(* Logix 5000 AddOnInstructionDefinition export EipIoDataMapping_GS30A_CM_EIP1; software revision 37.00 *)

ADD_ON_INSTRUCTION EipIoDataMapping_GS30A_CM_EIP1   (* revision 1.0, vendor Automationdirect.com *)
// This Add-On Instruction unpacks raw Input Data (T->O) from an array and maps this data into meaningful drive related status tags for the user. Likewise, the AOI also maps meaningful drive related command tags and packs the data into the raw Output Data (O->T) array.
// The purpose of the Add-On Instruction is to simplify the mapping (packing/unpacking) of the raw Input/Output Data. For operation of the drive, the user must provide their own logic.
// Revision note:
// Created in v37.00.00
// Version: 1.0
// - Initial version of the new Add-On Instruction format.
// 2025/06/27
VAR_IN_OUT
   mod_EipInputData : _0294:GS30A_CM_EIP1_E8411017:I:0; {required}   // Module defined using SINT data type
   mod_EipOutputData : _0294:GS30A_CM_EIP1_E771E08B:O:0; {required}   // Module defined using SINT data type
END_VAR
VAR_INPUT
   cmd_Run : BOOL; {visible}
   cmd_Stop : BOOL; {visible}
   cmd_Jog : BOOL; {visible}
   cmd_DirectionCommand : BOOL; {visible}   // False = Fwd; True = Rev
   cmd_NthAccelDecel : SINT; {visible}
   cmd_NthStepSpeedFrequency : SINT; {visible}
   cmd_EnableBitFunction_6_11 : BOOL; {visible}   // Enables the Nth Accel/Decel and Nth Step Speed Freq functionality
   cmd_FrequencyCommand : REAL; {visible}   // xx.xx Hz
   cmd_ExternalFaultTrigger : BOOL; {visible}
   cmd_ResetCommand : BOOL; {visible}
   cmd_ExternalInterruption : BOOL; {visible}
END_VAR
VAR_OUTPUT
   sts_WarningCode : SINT; {access Read Only, visible}
   sts_FaultCode : SINT; {access Read Only, visible}
   sts_Stop : BOOL; {access Read Only, visible}
   sts_DecelDuringStop : BOOL; {access Read Only, visible}
   sts_Standby : BOOL; {access Read Only, visible}
   sts_Run : BOOL; {access Read Only, visible}
   sts_Fwd : BOOL; {access Read Only, visible}
   sts_TransitioningRevToFwd : BOOL; {access Read Only, visible}
   sts_TransitioningFwdToRev : BOOL; {access Read Only, visible}
   sts_Rev : BOOL; {access Read Only, visible}
   sts_JogActive : BOOL; {access Read Only, visible}
   sts_FreqFromComm : BOOL; {access Read Only, visible}
   sts_FreqFromAnalogOrDiscrete : BOOL; {access Read Only, visible}
   sts_CommandFromCommKeypad : BOOL; {access Read Only, visible}
   sts_ParametersLocked : BOOL; {access Read Only, visible}
   sts_DriveStopped : BOOL; {access Read Only, visible}
   sts_DriveRunning : BOOL; {access Read Only, visible}
   sts_FreqCommand_PIDSetpoint : REAL; {access Read Only, visible}
   sts_OutputFrequency : REAL; {access Read Only, visible}   // xx.xx Hz
   sts_OutputCurrent : REAL; {access Read Only, visible}
   sts_DcBusVoltage : REAL; {access Read Only, visible}
   sts_OutputVoltage : REAL; {access Read Only, visible}   // xxx.x
   sts_MultiSpeed_PIDStepNumber : INT; {access Read Only, visible}
   sts_MaxOutputTorque : INT; {access Read Only, visible}
   sts_DigitalInputCounterValue : INT; {access Read Only, visible}
   sts_PowerFactorAngle : REAL; {access Read Only, visible}   // xxx.x degrees
   sts_OutputTorque : REAL; {access Read Only, visible}
   sts_ActualMotorSpeed : INT; {access Read Only, visible}   // xxxx RPM
   sts_EncoderFeedbackCounts : INT; {access None, visible}   // 0 to 65535
   sts_PulseCommandPositionCounts : INT; {access None, visible}   // 0 to 65535
   sts_PowerOutput : INT; {access Read Only, visible}   // xxxx kW (implied decimal)
END_VAR
VAR
   loc_iTemp : INT; {access None}   // Local INT for temporary data manipulation
END_VAR

ROUTINE Logic   (* ladder *)
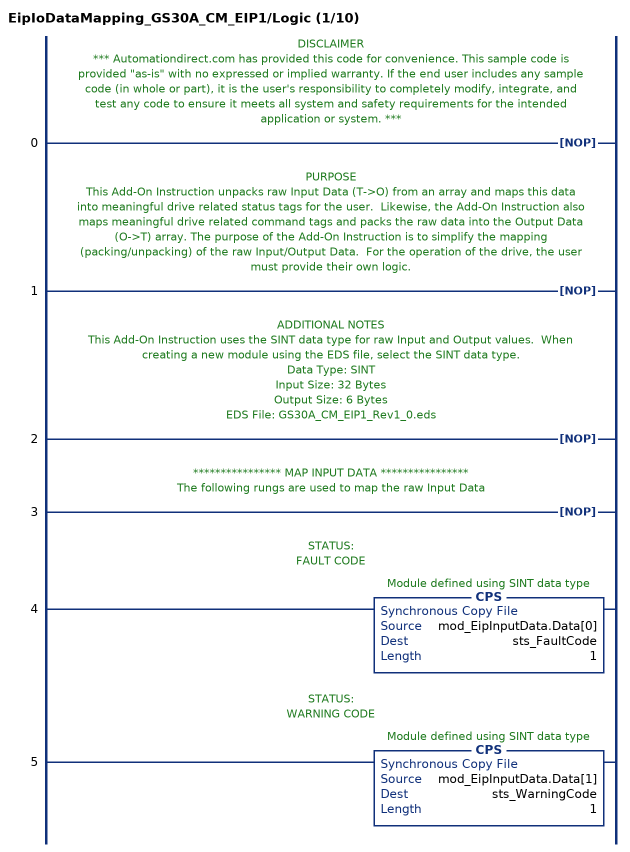
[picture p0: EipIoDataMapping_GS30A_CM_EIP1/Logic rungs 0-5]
   // DISCLAIMER
   // *** Automationdirect.com has provided this code for convenience. This sample code is provided "as-is" with no expressed or implied warranty. If the end user includes any sample code (in whole or part), it is the user's responsibility to completely modify, integrate, and test any code to ensure it meets all system and safety requirements for the intended application or system. ***
   0: NOP();
   // PURPOSE
   // This Add-On Instruction unpacks raw Input Data (T->O) from an array and maps this data into meaningful drive related status tags for the user.  Likewise, the Add-On Instruction also maps meaningful drive related command tags and packs the raw data into the Output Data (O->T) array. The purpose of the Add-On Instruction is to simplify the mapping (packing/unpacking) of the raw Input/Output Data.  For the operation of the drive, the user must provide their own logic.
   1: NOP();
   // ADDITIONAL NOTES
   // This Add-On Instruction uses the SINT data type for raw Input and Output values.  When creating a new module using the EDS file, select the SINT data type.
   // Data Type: SINT
   // Input Size: 32 Bytes
   // Output Size: 6 Bytes
   // EDS File: GS30A_CM_EIP1_Rev1_0.eds
   2: NOP();
   // **************** MAP INPUT DATA ****************
   // The following rungs are used to map the raw Input Data
   3: NOP();
   // STATUS:
   // FAULT CODE
   4: CPS(mod_EipInputData.Data[0],sts_FaultCode,1);
   // STATUS:
   // WARNING CODE
   5: CPS(mod_EipInputData.Data[1],sts_WarningCode,1);
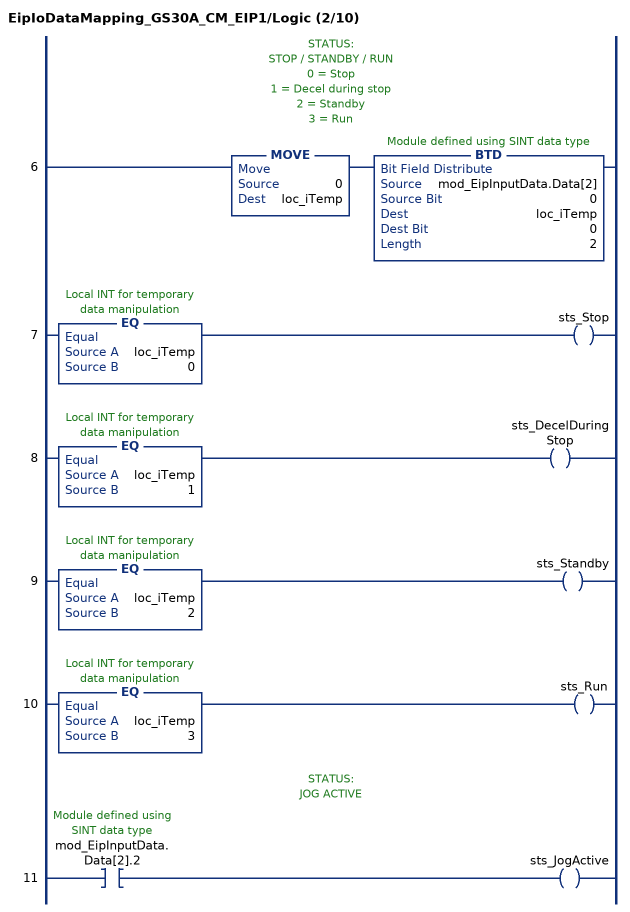
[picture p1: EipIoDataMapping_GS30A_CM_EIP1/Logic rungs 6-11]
   // STATUS:
   // STOP / STANDBY / RUN
   // 0 = Stop
   // 1 = Decel during stop
   // 2 = Standby
   // 3 = Run
   6: MOVE(0,loc_iTemp)BTD(mod_EipInputData.Data[2],0,loc_iTemp,0,2);
   7: EQ(loc_iTemp,0)OTE(sts_Stop);
   8: EQ(loc_iTemp,1)OTE(sts_DecelDuringStop);
   9: EQ(loc_iTemp,2)OTE(sts_Standby);
   10: EQ(loc_iTemp,3)OTE(sts_Run);
   // STATUS:
   // JOG ACTIVE
   11: XIC(mod_EipInputData.Data[2].2)OTE(sts_JogActive);
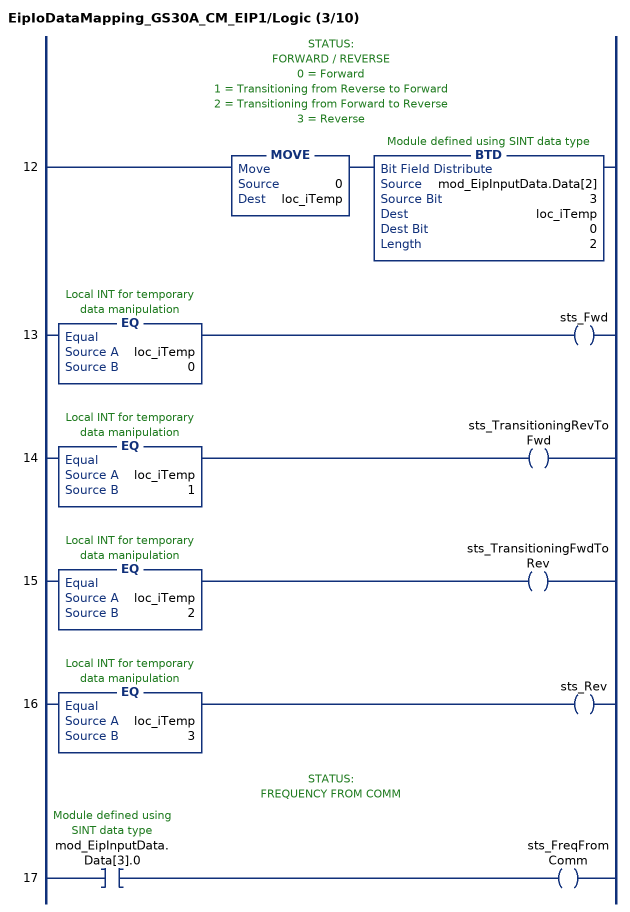
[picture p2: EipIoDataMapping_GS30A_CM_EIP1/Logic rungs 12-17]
   // STATUS:
   // FORWARD / REVERSE
   // 0 = Forward
   // 1 = Transitioning from Reverse to Forward
   // 2 = Transitioning from Forward to Reverse
   // 3 = Reverse
   12: MOVE(0,loc_iTemp)BTD(mod_EipInputData.Data[2],3,loc_iTemp,0,2);
   13: EQ(loc_iTemp,0)OTE(sts_Fwd);
   14: EQ(loc_iTemp,1)OTE(sts_TransitioningRevToFwd);
   15: EQ(loc_iTemp,2)OTE(sts_TransitioningFwdToRev);
   16: EQ(loc_iTemp,3)OTE(sts_Rev);
   // STATUS:
   // FREQUENCY FROM COMM
   17: XIC(mod_EipInputData.Data[3].0)OTE(sts_FreqFromComm);
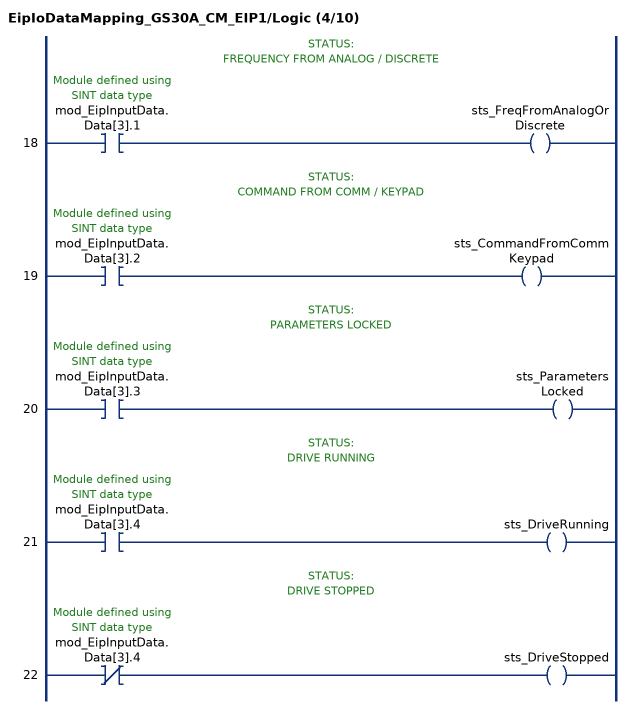
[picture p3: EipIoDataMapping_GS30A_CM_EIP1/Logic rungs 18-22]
   // STATUS:
   // FREQUENCY FROM ANALOG / DISCRETE
   18: XIC(mod_EipInputData.Data[3].1)OTE(sts_FreqFromAnalogOrDiscrete);
   // STATUS:
   // COMMAND FROM COMM / KEYPAD
   19: XIC(mod_EipInputData.Data[3].2)OTE(sts_CommandFromCommKeypad);
   // STATUS:
   // PARAMETERS LOCKED
   20: XIC(mod_EipInputData.Data[3].3)OTE(sts_ParametersLocked);
   // STATUS:
   // DRIVE RUNNING
   21: XIC(mod_EipInputData.Data[3].4)OTE(sts_DriveRunning);
   // STATUS:
   // DRIVE STOPPED
   22: XIO(mod_EipInputData.Data[3].4)OTE(sts_DriveStopped);
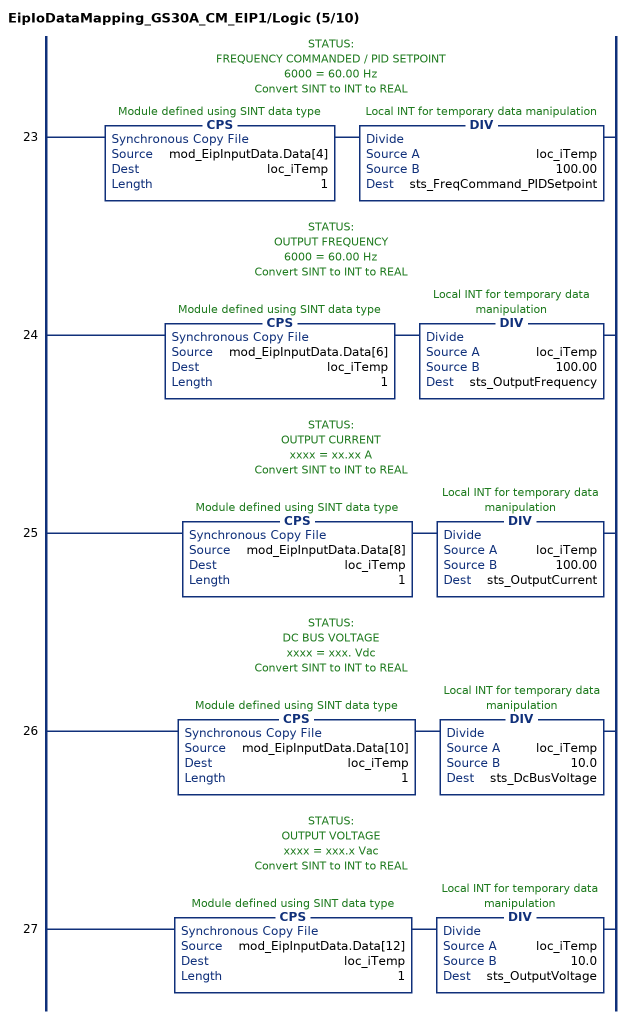
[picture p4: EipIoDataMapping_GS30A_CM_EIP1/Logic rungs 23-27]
   // STATUS:
   // FREQUENCY COMMANDED / PID SETPOINT
   // 6000 = 60.00 Hz
   // Convert SINT to INT to REAL
   23: CPS(mod_EipInputData.Data[4],loc_iTemp,1)DIV(loc_iTemp,100.00,sts_FreqCommand_PIDSetpoint);
   // STATUS:
   // OUTPUT FREQUENCY
   // 6000 = 60.00 Hz
   // Convert SINT to INT to REAL
   24: CPS(mod_EipInputData.Data[6],loc_iTemp,1)DIV(loc_iTemp,100.00,sts_OutputFrequency);
   // STATUS:
   // OUTPUT CURRENT
   // xxxx = xx.xx A
   // Convert SINT to INT to REAL
   25: CPS(mod_EipInputData.Data[8],loc_iTemp,1)DIV(loc_iTemp,100.00,sts_OutputCurrent);
   // STATUS:
   // DC BUS VOLTAGE
   // xxxx = xxx. Vdc
   // Convert SINT to INT to REAL
   26: CPS(mod_EipInputData.Data[10],loc_iTemp,1)DIV(loc_iTemp,10.0,sts_DcBusVoltage);
   // STATUS:
   // OUTPUT VOLTAGE
   // xxxx = xxx.x Vac
   // Convert SINT to INT to REAL
   27: CPS(mod_EipInputData.Data[12],loc_iTemp,1)DIV(loc_iTemp,10.0,sts_OutputVoltage);
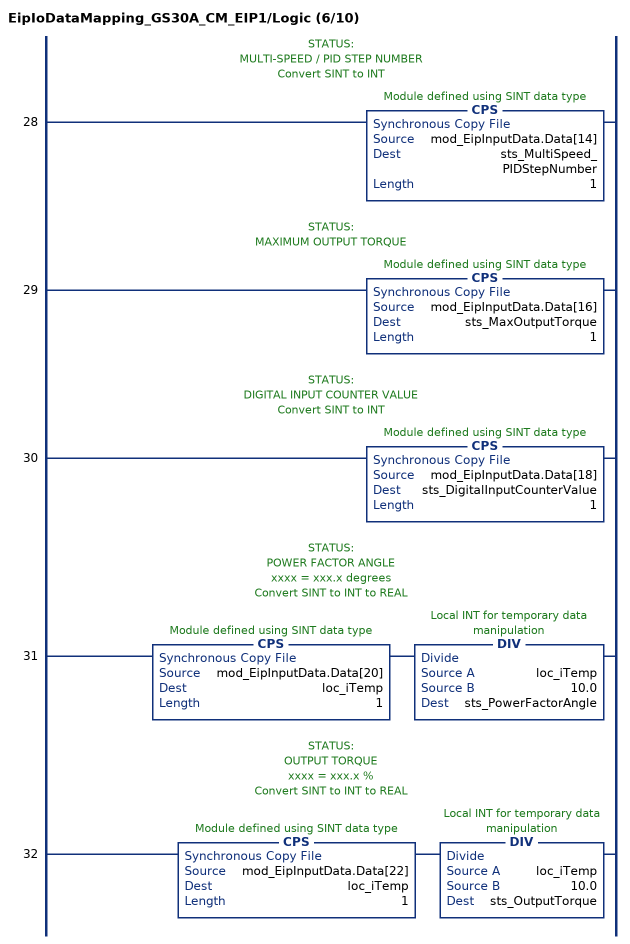
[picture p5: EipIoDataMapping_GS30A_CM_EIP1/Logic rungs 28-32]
   // STATUS:
   // MULTI-SPEED / PID STEP NUMBER
   // Convert SINT to INT
   28: CPS(mod_EipInputData.Data[14],sts_MultiSpeed_PIDStepNumber,1);
   // STATUS:
   // MAXIMUM OUTPUT TORQUE
   29: CPS(mod_EipInputData.Data[16],sts_MaxOutputTorque,1);
   // STATUS:
   // DIGITAL INPUT COUNTER VALUE
   // Convert SINT to INT
   30: CPS(mod_EipInputData.Data[18],sts_DigitalInputCounterValue,1);
   // STATUS:
   // POWER FACTOR ANGLE
   // xxxx = xxx.x degrees
   // Convert SINT to INT to REAL
   31: CPS(mod_EipInputData.Data[20],loc_iTemp,1)DIV(loc_iTemp,10.0,sts_PowerFactorAngle);
   // STATUS:
   // OUTPUT TORQUE
   // xxxx = xxx.x %
   // Convert SINT to INT to REAL
   32: CPS(mod_EipInputData.Data[22],loc_iTemp,1)DIV(loc_iTemp,10.0,sts_OutputTorque);
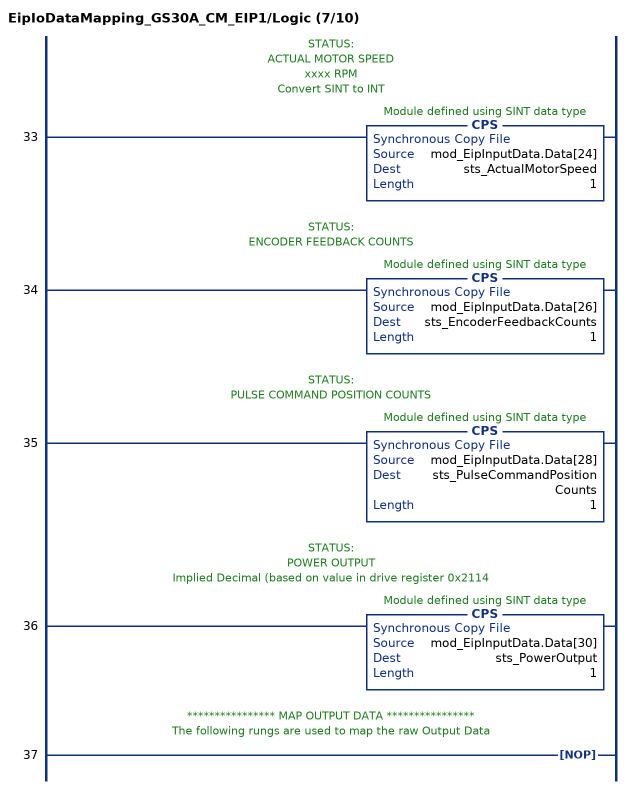
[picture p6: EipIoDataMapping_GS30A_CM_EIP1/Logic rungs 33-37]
   // STATUS:
   // ACTUAL MOTOR SPEED
   // xxxx RPM
   // Convert SINT to INT
   33: CPS(mod_EipInputData.Data[24],sts_ActualMotorSpeed,1);
   // STATUS:
   // ENCODER FEEDBACK COUNTS
   34: CPS(mod_EipInputData.Data[26],sts_EncoderFeedbackCounts,1);
   // STATUS:
   // PULSE COMMAND POSITION COUNTS
   35: CPS(mod_EipInputData.Data[28],sts_PulseCommandPositionCounts,1);
   // STATUS:
   // POWER OUTPUT
   // Implied Decimal (based on value in drive register 0x2114
   36: CPS(mod_EipInputData.Data[30],sts_PowerOutput,1);
   // **************** MAP OUTPUT DATA ****************
   // The following rungs are used to map the raw Output Data
   37: NOP();
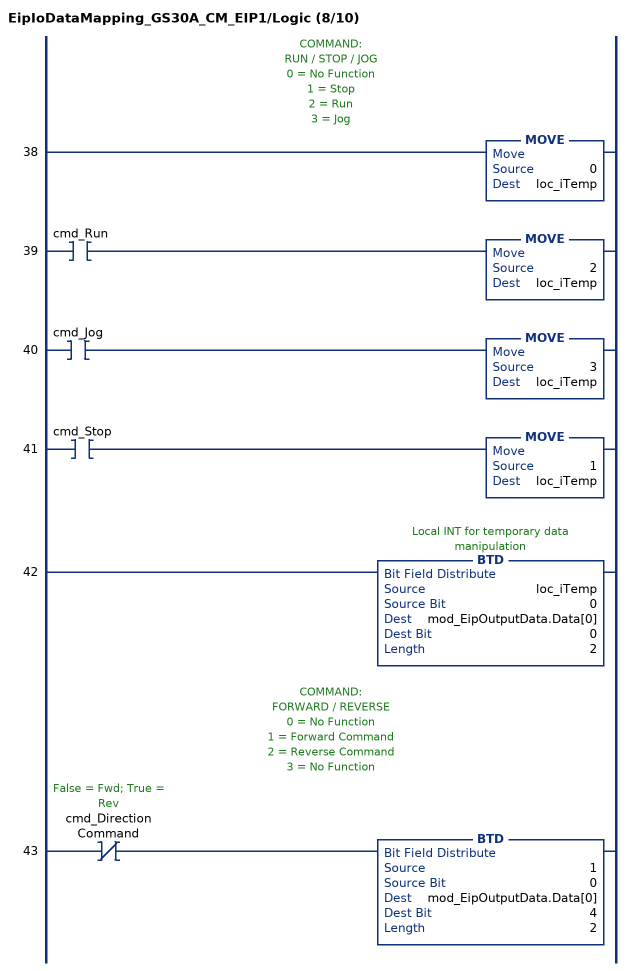
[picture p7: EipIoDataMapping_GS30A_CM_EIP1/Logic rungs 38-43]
   // COMMAND:
   // RUN / STOP / JOG
   // 0 = No Function
   // 1 = Stop
   // 2 = Run
   // 3 = Jog
   38: MOVE(0,loc_iTemp);
   39: XIC(cmd_Run)MOVE(2,loc_iTemp);
   40: XIC(cmd_Jog)MOVE(3,loc_iTemp);
   41: XIC(cmd_Stop)MOVE(1,loc_iTemp);
   42: BTD(loc_iTemp,0,mod_EipOutputData.Data[0],0,2);
   // COMMAND:
   // FORWARD / REVERSE
   // 0 = No Function
   // 1 = Forward Command
   // 2 = Reverse Command
   // 3 = No Function
   43: XIO(cmd_DirectionCommand)BTD(1,0,mod_EipOutputData.Data[0],4,2);
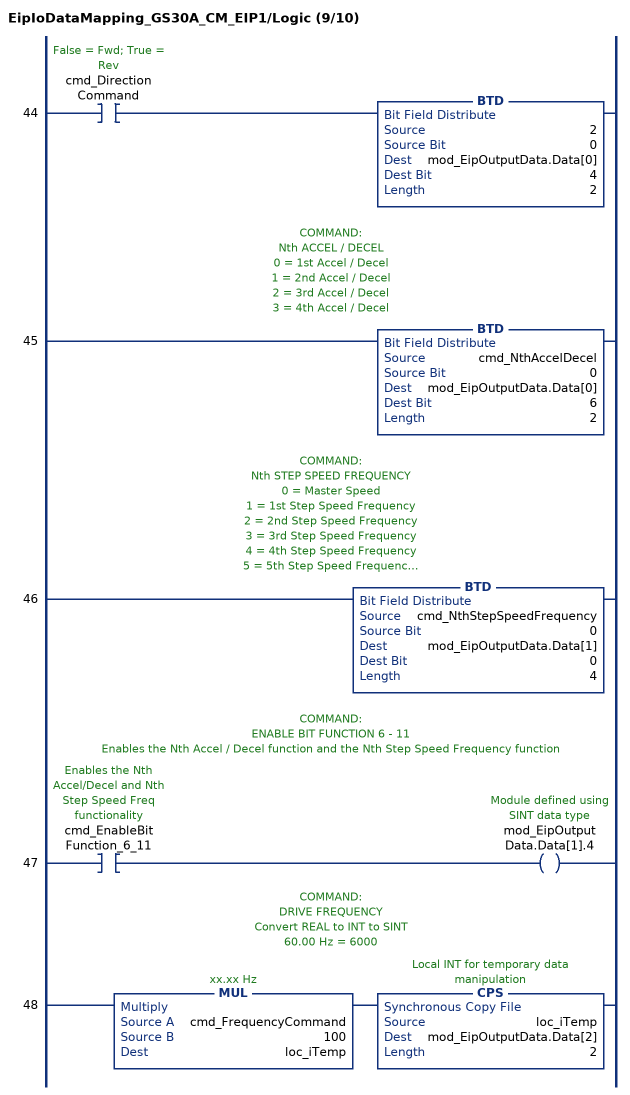
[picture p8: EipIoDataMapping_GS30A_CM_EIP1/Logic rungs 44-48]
   44: XIC(cmd_DirectionCommand)BTD(2,0,mod_EipOutputData.Data[0],4,2);
   // COMMAND:
   // Nth ACCEL / DECEL
   // 0 = 1st Accel / Decel
   // 1 = 2nd Accel / Decel
   // 2 = 3rd Accel / Decel
   // 3 = 4th Accel / Decel
   45: BTD(cmd_NthAccelDecel,0,mod_EipOutputData.Data[0],6,2);
   // COMMAND:
   // Nth STEP SPEED FREQUENCY
   // 0 = Master Speed
   // 1 = 1st Step Speed Frequency
   // 2 = 2nd Step Speed Frequency
   // 3 = 3rd Step Speed Frequency
   // 4 = 4th Step Speed Frequency
   // 5 = 5th Step Speed Frequency
   // 6 = 6th Step Speed Frequency
   // 7 = 7th Step Speed Frequency
   // 8 = 8th Step Speed Frequency
   // 9 = 9th Step Speed Frequency
   // 10 = 10th Step Speed Frequency
   // 11 = 11th Step Speed Frequency
   // 12 = 12th Step Speed Frequency
   // 13 = 13th Step Speed Frequency
   // 14 = 14th Step Speed Frequency
   // 15 = 15th Step Speed Frequency
   46: BTD(cmd_NthStepSpeedFrequency,0,mod_EipOutputData.Data[1],0,4);
   // COMMAND:
   // ENABLE BIT FUNCTION 6 - 11
   // Enables the Nth Accel / Decel function and the Nth Step Speed Frequency function
   47: XIC(cmd_EnableBitFunction_6_11)OTE(mod_EipOutputData.Data[1].4);
   // COMMAND:
   // DRIVE FREQUENCY
   // Convert REAL to INT to SINT
   // 60.00 Hz = 6000
   48: MUL(cmd_FrequencyCommand,100,loc_iTemp)CPS(loc_iTemp,mod_EipOutputData.Data[2],2);
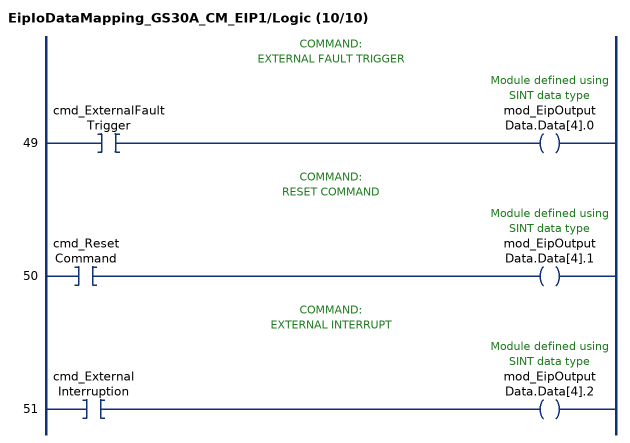
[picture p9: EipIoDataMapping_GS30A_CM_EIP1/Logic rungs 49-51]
   // COMMAND:
   // EXTERNAL FAULT TRIGGER
   49: XIC(cmd_ExternalFaultTrigger)OTE(mod_EipOutputData.Data[4].0);
   // COMMAND:
   // RESET COMMAND
   50: XIC(cmd_ResetCommand)OTE(mod_EipOutputData.Data[4].1);
   // COMMAND:
   // EXTERNAL INTERRUPT
   51: XIC(cmd_ExternalInterruption)OTE(mod_EipOutputData.Data[4].2);
END_ROUTINE
END_ADD_ON_INSTRUCTION
